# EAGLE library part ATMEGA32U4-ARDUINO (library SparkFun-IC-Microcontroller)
Atmel MCU, 32KByte Atmel 44-pin 8-bit Microcontroller with 32KBytes of ISP Flash and USB Controller Datasheet SparkFun Products LilyPad Arduino USB - ATmega32U4 Board (DEV-12049) Pro Micro - 5V/16MHz (DEV-12640) Pro Micro - 3.3V/8MHz (DEV-12587) Fio v3 - ATmega32U4 (DEV-11520) Qduino Mini (DEV-13614) Makey Makey - Standard Kit (WIG-11511) Makey Makey Deluxe Kit (WIG-11519)
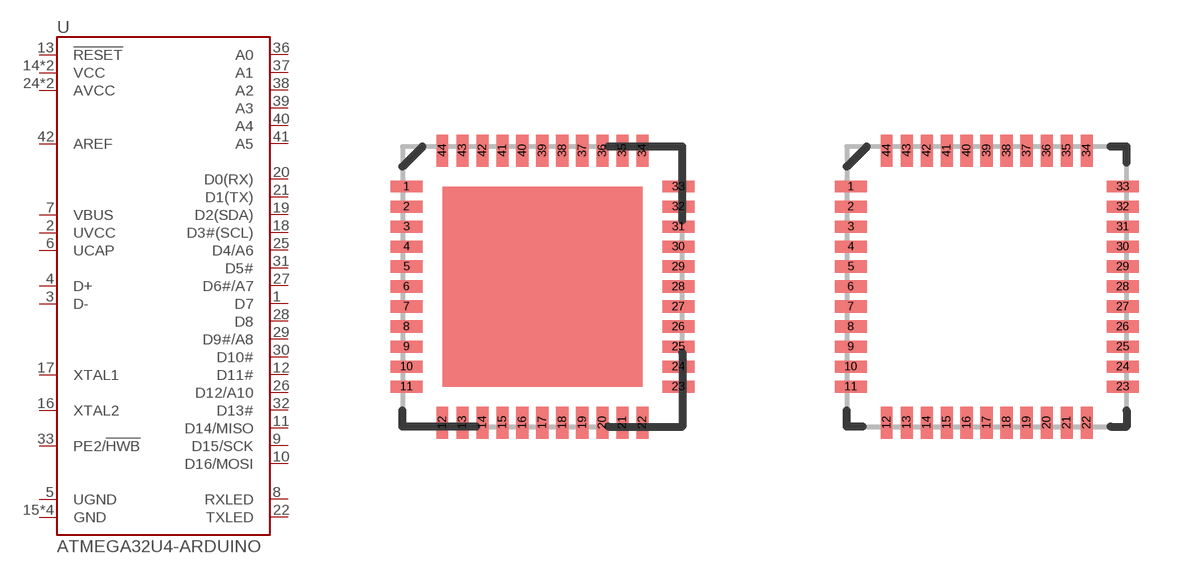
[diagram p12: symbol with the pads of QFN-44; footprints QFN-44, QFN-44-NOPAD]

Designator prefix U

## ATMEGA32U4-ARDUINOQFN (PROD_ID: IC-10828; VALUE: 32U4)  [QFN-44]
1  D7
2  UVCC
3  D-
4  D+
5  UGND
6  UCAP
7  VBUS
8  RXLED
9  D15/SCK
10  D16/MOSI
11  D14/MISO
12  D11#
13  !RESET
14  VCC
15  GND
16  XTAL2
17  XTAL1
18  D3#(SCL)
19  D2(SDA)
20  D0(RX)
21  D1(TX)
22  TXLED
23  GND
24  AVCC
25  D4/A6
26  D12/A10
27  D6#/A7
28  D8
29  D9#/A8
30  D10#
31  D5#
32  D13#
33  PE2/!HWB
34  VCC
35  GND
36  A0
37  A1
38  A2
39  A3
40  A4
41  A5
42  AREF
43  GND
44  AVCC

## ATMEGA32U4-ARDUINOQFN2 (PROD_ID: IC-10828; VALUE: 32U4)  [QFN-44-NOPAD]
Pads as for QFN-44

## ATMEGA32U4-ARDUINO1:1 (PROD_ID: IC-10828; VALUE: 32U4)  [QFN-44-NOPAD_1:1]
Pads as for QFN-44

## ATMEGA32U4-ARDUINO1:1-LESS_PASTE (PROD_ID: IC-10828; VALUE: 32U4)  [QFN-44-NOPAD_1:1-LESS_PASTE]
Pads as for QFN-44

## ATMEGA32U4-ARDUINOTQFP-44 (PROD_ID: IC-11161; VALUE: 32U4)  [TQFP44]
Pads as for QFN-44

## Footprint QFN-44 (pad centres in mm)
smd 0.8 x 0.3: 1 -3.4,2.5; 2 -3.4,2; 3 -3.4,1.5; 4 -3.4,1; 5 -3.4,0.5; 6 -3.4,0; 7 -3.4,-0.5; 8 -3.4,-1; 9 -3.4,-1.5; 10 -3.4,-2; 11 -3.4,-2.5; 23 3.4,-2.5; 24 3.4,-2; 25 3.4,-1.5; 26 3.4,-1; 27 3.4,-0.5; 28 3.4,0; 29 3.4,0.5; 30 3.4,1; 31 3.4,1.5; 32 3.4,2; 33 3.4,2.5
smd 0.3 x 0.8: 12 -2.5,-3.4; 13 -2,-3.4; 14 -1.5,-3.4; 15 -1,-3.4; 16 -0.5,-3.4; 17 0,-3.4; 18 0.5,-3.4; 19 1,-3.4; 20 1.5,-3.4; 21 2,-3.4; 22 2.5,-3.4; 34 2.5,3.4; 35 2,3.4; 36 1.5,3.4; 37 1,3.4; 38 0.5,3.4; 39 0,3.4; 40 -0.5,3.4; 41 -1,3.4; 42 -1.5,3.4; 43 -2,3.4; 44 -2.5,3.4

## Footprint QFN-44-NOPAD (pad centres in mm)
smd 0.8 x 0.3: 1 -3.4,2.5; 2 -3.4,2; 3 -3.4,1.5; 4 -3.4,1; 5 -3.4,0.5; 6 -3.4,0; 7 -3.4,-0.5; 8 -3.4,-1; 9 -3.4,-1.5; 10 -3.4,-2; 11 -3.4,-2.5; 23 3.4,-2.5; 24 3.4,-2; 25 3.4,-1.5; 26 3.4,-1; 27 3.4,-0.5; 28 3.4,0; 29 3.4,0.5; 30 3.4,1; 31 3.4,1.5; 32 3.4,2; 33 3.4,2.5
smd 0.3 x 0.8: 12 -2.5,-3.4; 13 -2,-3.4; 14 -1.5,-3.4; 15 -1,-3.4; 16 -0.5,-3.4; 17 0,-3.4; 18 0.5,-3.4; 19 1,-3.4; 20 1.5,-3.4; 21 2,-3.4; 22 2.5,-3.4; 34 2.5,3.4; 35 2,3.4; 36 1.5,3.4; 37 1,3.4; 38 0.5,3.4; 39 0,3.4; 40 -0.5,3.4; 41 -1,3.4; 42 -1.5,3.4; 43 -2,3.4; 44 -2.5,3.4

## Footprint QFN-44-NOPAD_1:1 (pad centres in mm)
smd 0.8 x 0.3: 1 -3.337,2.458; 2 -3.337,1.958; 3 -3.337,1.479; 4 -3.337,0.979; 5 -3.337,0.5; 6 -3.337,0; 7 -3.337,-0.5; 8 -3.337,-0.979; 9 -3.337,-1.479; 10 -3.337,-1.958; 11 -3.337,-2.458; 23 3.337,-2.458; 24 3.337,-1.958; 25 3.337,-1.479; 26 3.337,-0.979; 27 3.337,-0.5; 28 3.337,0; 29 3.337,0.5; 30 3.337,0.979; 31 3.337,1.479; 32 3.337,1.958; 33 3.337,2.458
smd 0.3 x 0.8: 12 -2.458,-3.337; 13 -1.958,-3.337; 14 -1.479,-3.337; 15 -0.979,-3.337; 16 -0.5,-3.337; 17 0,-3.337; 18 0.5,-3.337; 19 0.979,-3.337; 20 1.479,-3.337; 21 1.958,-3.337; 22 2.458,-3.337; 34 2.458,3.337; 35 1.958,3.337; 36 1.479,3.337; 37 0.979,3.337; 38 0.5,3.337; 39 0,3.337; 40 -0.5,3.337; 41 -0.979,3.337; 42 -1.479,3.337; 43 -1.958,3.337; 44 -2.458,3.337

## Footprint QFN-44-NOPAD_1:1-LESS_PASTE (pad centres in mm)
smd 0.8 x 0.3: 1 -3.337,2.458; 2 -3.337,1.958; 3 -3.337,1.479; 4 -3.337,0.979; 5 -3.337,0.5; 6 -3.337,0; 7 -3.337,-0.5; 8 -3.337,-0.979; 9 -3.337,-1.479; 10 -3.337,-1.958; 11 -3.337,-2.458; 23 3.337,-2.458; 24 3.337,-1.958; 25 3.337,-1.479; 26 3.337,-0.979; 27 3.337,-0.5; 28 3.337,0; 29 3.337,0.5; 30 3.337,0.979; 31 3.337,1.479; 32 3.337,1.958; 33 3.337,2.458
smd 0.3 x 0.8: 12 -2.458,-3.337; 13 -1.958,-3.337; 14 -1.479,-3.337; 15 -0.979,-3.337; 16 -0.5,-3.337; 17 0,-3.337; 18 0.5,-3.337; 19 0.979,-3.337; 20 1.479,-3.337; 21 1.958,-3.337; 22 2.458,-3.337; 34 2.458,3.337; 35 1.958,3.337; 36 1.479,3.337; 37 0.979,3.337; 38 0.5,3.337; 39 0,3.337; 40 -0.5,3.337; 41 -0.979,3.337; 42 -1.479,3.337; 43 -1.958,3.337; 44 -2.458,3.337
